| IBIS file 71v3578Z_bg.ibs created by s2ibis2 version 1.1
| North Carolina State University Electronics Research Laboratory  1995
[IBIS ver]   2.1
[File name]   71v3578z_bg.ibs
[File Rev]   1.1
[Date]   8/16/00
[Source]   Integrated Device Technology, Inc.
[Notes]   1. Temperatures: typ=25C, min=70C, max=0C 2. Cemos10_3v
   process. 3. Ramp rates based on 50 ohm load.
[Copyright]   Copyright 2000, Integrated Device Technology, Inc. Integrated
   Device Technology, Inc. ("IDT") hereby grants the user of this
   IBIS model a non-exclusive, nontransferable license to use
   this IBIS model under the following terms. The user is granted
   this license only to use the IBIS model and is not granted
   rights to sell, copy (except as needed to run the IBIS model),
   rent, lease or sub-license the IBIS model in whole or in part,
   or in modified form to anyone. The User may modify the IBIS
   model to suit its specific applications, but rights to
   derivative works and such modifications shall belong to IDT.
   This IBIS model is provided on an AS IS" basis and IDT makes
   absolutely no warranty with respect to the information
   contained herein. IDT DISCLAIMS AND CUSTOMER WAIVES ALL
   WARRANTIES, EXPRESS AND IMPLIED, INCLUDING WARRANTIES OF
   MERCHANTABILITY AND FITNESS FOR A PARTICULAR PURPOSE. THE
   ENTIRE RISK AS TO QUALITY AND PERFORMANCE IS WITH THE USER
   ACCORDINGLY, IN NO EVENT SHALL IDT BE LIABLE FOR ANY DIRECT OR
   INDIRECT DAMAGES, WHETHER IN CONTRACT OR TORT, INCLUDING ANY
   LOST PROFITS OR OTHER INCIDENTAL, CONSEQUENTIAL, EXEMPLARY, OR
   PUNITIVE DAMAGES ARISING OUT OF THE USE OR APPLICATION OF THE
   IBIS model. Further, IDT reserves the right to make changes
   without notice to any product herein to improve reliability,
   function, or design. IDT does not convey any license under
   patent rights or any other intellectual property rights,
   including those of third parties. IDT is not obligated to
   provide maintenance or support for the licensed IBIS model.
|   Component idt71V3578Z
[Component]   idt71V3578Z
[Manufacturer]   Integrated Device Technology
|   This component uses the 119 BGA package (BG)
[Package]
| variable   typ   min   max
R_pkg   328m   103m   556m
L_pkg   5.4nH   2.8nH   20.4nH
C_pkg   2.1pF   1.06pF   4.4pF
[Pin]  signal_name   model_name   R_pin   L_pin   C_pin
A1   VDDQ   POWER
A2   A6   INPAD_71V3578Z
A3   A4   INPAD_71V3578Z
A4   NADSP   INPAD_71V3578Z
A5   A8   INPAD_71V3578Z
A6   A16   INPAD_71V3578Z
A7   VDDQ   POWER
B1   NC   NC
B2   CS0   INPAD_71V3578Z
B3   A3   INPAD_71V3578Z
B4   NADSC   INPAD_71V3578Z
B5   A9   INPAD_71V3578Z
B6   NCS1   INPAD_71V3578Z
B7   NC   NC
C1   NC   NC
C2   A7   INPAD_71V3578Z
C3   A2   INPAD_71V3578Z
C4   VDD   POWER
C5   A13   INPAD_71V3578Z
C6   A17   INPAD_71V3578Z
C7   NC   NC
D1   IO8   IOPAD3578Z
D2   NC   NC
D3   VSS   GND
D4   NC   NC
D5   VSS   GND
D6   IO7   IOPAD3578Z
D7   NC   NC
E1   NC   NC
E2   IO9   IOPAD3578Z
E3   VSS   GND
E4   NCE   INPAD_71V3578Z
E5   VSS   GND
E6   NC   NC
E7   IO6   IOPAD3578Z
F1   VDDQ   POWER
F2   NC   NC
F3   VSS   GND
F4   NOE   INPAD_71V3578Z
F5   VSS   GND
F6   IO5   IOPAD3578Z
F7   VDDQ   POWER
G1   NC   NC
G2   IO10   IOPAD3578Z
G3   NBW2   INPAD_71V3578Z
G4   NADV   INPAD_71V3578Z
G5   VSS   GND
G6   NC   NC
G7   IO4   IOPAD3578Z
H1   IO11   IOPAD3578Z
H2   NC   NC
H3   VSS   GND
H4   NGW   INPAD_71V3578Z
H5   VSS   GND
H6   IO3   IOPAD3578Z
H7   NC   NC
J1   VDDQ   POWER
J2   VDD   POWER
J3   NC   NC
J4   VDD   POWER
J5   NC   NC
J6   VDD   POWER
J7   VDDQ   POWER
K1   NC   NC
K2   IO12   IOPAD3578Z
K3   VSS   GND
K4   CLK   INCLK_71V3578Z
K5   VSS   GND
K6   NC   NC
K7   IO2   IOPAD3578Z
L1   IO13   IOPAD3578Z
L2   NC   NC
L3   VSS   GND
L4   NC   NC
L5   NBW1   INPAD_71V3578Z
L6   IO1   IOPAD3578Z
L7   NC   NC
M1   VDDQ   POWER
M2   IO14   IOPAD3578Z
M3   VSS   GND
M4   NBWE   INPAD_71V3578Z
M5   VSS   GND
M6   NC   NC
M7   VDDQ   POWER
N1   IO15   IOPAD3578Z
N2   NC   NC
N3   VSS   GND
N4   A1   INPAD_71V3578Z
N5   VSS   GND
N6   IO0   IOPAD3578Z
N7   NC   NC
P1   NC   NC
P2   IOP2   IOPAD3578Z
P3   VSS   GND
P4   A0   INPAD_71V3578Z
P5   VSS   GND
P6   NC   NC
P7   IOP1   IOPAD3578Z
R1   NC   NC
R2   A5   INPAD_71V3578Z
R3   NLBO   INPAD_71V3578Z
R4   VDD   POWER
R5   VDD   POWER
R6   A12   INPAD_71V3578Z
R7   NC   NC
T1   NC   NC
T2   A10   INPAD_71V3578Z
T3   A15   INPAD_71V3578Z
T4   NC   NC
T5   A14   INPAD_71V3578Z
T6   A11   INPAD_71V3578Z
T7   ZZ   INPAD_71V3578Z
U1   VDDQ   POWER
U2   NC   NC
U3   NC   NC
U4   NC   NC
U5   NC   NC
U6   NC   NC
U7   VDDQ   POWER
U70   GNDQ   GND
| IOIN IOIN   dummy_model
| OC   OC   dummy_model
| IN   IN   dummy_model
| CLK  CLK   dummy_model
[Pin Mapping]  pulldown_ref   pullup_ref   gnd_clamp_ref   power_clamp_ref
A1   NC   EXTVDDQ
A2   EXTGNDQ   EXTVDDQ   EXTGND   EXTVDD
A3   EXTGNDQ   EXTVDDQ   EXTGND   EXTVDD
A4   EXTGNDQ   EXTVDDQ   EXTGND   EXTVDD
A5   EXTGNDQ   EXTVDDQ   EXTGND   EXTVDD
A6   EXTGNDQ   EXTVDDQ   EXTGND   EXTVDD
A7   NC   EXTVDDQ
B1   NC   NC   NC   NC
B2   EXTGNDQ   EXTVDDQ   EXTGND   EXTVDD
B3   EXTGNDQ   EXTVDDQ   EXTGND   EXTVDD
B4   EXTGNDQ   EXTVDDQ   EXTGND   EXTVDD
B5   EXTGNDQ   EXTVDDQ   EXTGND   EXTVDD
B6   EXTGNDQ   EXTVDDQ   EXTGND   EXTVDD
B7   NC   NC   NC   NC
C1   NC   NC   NC   NC
C2   EXTGNDQ   EXTVDDQ   EXTGND   EXTVDD
C3   EXTGNDQ   EXTVDDQ   EXTGND   EXTVDD
C4   NC   EXTVDD
C5   EXTGNDQ   EXTVDDQ   EXTGND   EXTVDD
C6   EXTGNDQ   EXTVDDQ   EXTGND   EXTVDD
C7   NC   NC   NC   NC
D1   EXTGNDQ   EXTVDDQ   EXTGND   EXTVDD
D2   NC   NC   NC   NC
D3   EXTGND   NC
D4   NC   NC   NC   NC
D5   EXTGND   NC
D6   EXTGNDQ   EXTVDDQ   EXTGND   EXTVDD
D7   NC   NC   NC   NC
E1   NC   NC   NC   NC
E2   EXTGNDQ   EXTVDDQ   EXTGND   EXTVDD
E3   EXTGND   NC
E4   EXTGNDQ   EXTVDDQ   EXTGND   EXTVDD
E5   EXTGND   NC
E6   NC   NC   NC   NC
E7   EXTGNDQ   EXTVDDQ   EXTGND   EXTVDD
F1   NC   EXTVDDQ
F2   NC   NC   NC   NC
F3   EXTGND   NC
F4   EXTGNDQ   EXTVDDQ   EXTGND   EXTVDD
F5   EXTGND   NC
F6   EXTGNDQ   EXTVDDQ   EXTGND   EXTVDD
F7   NC   EXTVDDQ
G1   NC   NC   NC   NC
G2   EXTGNDQ   EXTVDDQ   EXTGND   EXTVDD
G3   EXTGNDQ   EXTVDDQ   EXTGND   EXTVDD
G4   EXTGNDQ   EXTVDDQ   EXTGND   EXTVDD
G5   EXTGND   NC
G6   NC   NC   NC   NC
G7   EXTGNDQ   EXTVDDQ   EXTGND   EXTVDD
H1   EXTGNDQ   EXTVDDQ   EXTGND   EXTVDD
H2   NC   NC   NC   NC
H3   EXTGND   NC
H4   EXTGNDQ   EXTVDDQ   EXTGND   EXTVDD
H5   EXTGND   NC
H6   EXTGNDQ   EXTVDDQ   EXTGND   EXTVDD
H7   NC   NC   NC   NC
J1   NC   EXTVDDQ
J2   NC   EXTVDD
J3   NC   NC   NC   NC
J4   NC   EXTVDD
J5   NC   NC   NC   NC
J6   NC   EXTVDD
J7   NC   EXTVDDQ
K1   NC   NC   NC   NC
K2   EXTGNDQ   EXTVDDQ   EXTGND   EXTVDD
K3   EXTGND   NC
K4   EXTGNDQ   EXTVDDQ   EXTGND   EXTVDD
K5   EXTGND   NC
K6   NC   NC   NC   NC
K7   EXTGNDQ   EXTVDDQ   EXTGND   EXTVDD
L1   EXTGNDQ   EXTVDDQ   EXTGND   EXTVDD
L2   NC   NC   NC   NC
L3   EXTGND   NC
L4   NC   NC   NC   NC
L5   EXTGNDQ   EXTVDDQ   EXTGND   EXTVDD
L6   EXTGNDQ   EXTVDDQ   EXTGND   EXTVDD
L7   NC   NC   NC   NC
M1   NC   EXTVDDQ
M2   EXTGNDQ   EXTVDDQ   EXTGND   EXTVDD
M3   EXTGND   NC
M4   EXTGNDQ   EXTVDDQ   EXTGND   EXTVDD
M5   EXTGND   NC
M6   NC   NC   NC   NC
M7   NC   EXTVDDQ
N1   EXTGNDQ   EXTVDDQ   EXTGND   EXTVDD
N2   NC   NC   NC   NC
N3   EXTGND   NC
N4   EXTGNDQ   EXTVDDQ   EXTGND   EXTVDD
N5   EXTGND   NC
N6   EXTGNDQ   EXTVDDQ   EXTGND   EXTVDD
N7   NC   NC   NC   NC
P1   NC   NC   NC   NC
P2   EXTGNDQ   EXTVDDQ   EXTGND   EXTVDD
P3   EXTGND   NC
P4   EXTGNDQ   EXTVDDQ   EXTGND   EXTVDD
P5   EXTGND   NC
P6   NC   NC   NC   NC
P7   EXTGNDQ   EXTVDDQ   EXTGND   EXTVDD
R1   NC   NC   NC   NC
R2   EXTGNDQ   EXTVDDQ   EXTGND   EXTVDD
R3   EXTGNDQ   EXTVDDQ   EXTGND   EXTVDD
R4   NC   EXTVDD
R5   NC   EXTVDD
R6   EXTGNDQ   EXTVDDQ   EXTGND   EXTVDD
R7   NC   NC   NC   NC
T1   NC   NC   NC   NC
T2   NC   NC   NC   NC
T3   EXTGNDQ   EXTVDDQ   EXTGND   EXTVDD
T4   NC   NC   NC   NC
T5   EXTGNDQ   EXTVDDQ   EXTGND   EXTVDD
T6   NC   NC   NC   NC
T7   EXTGNDQ   EXTVDDQ   EXTGND   EXTVDD
U1   NC   EXTVDDQ
U2   NC   NC   NC   NC
U3   NC   NC   NC   NC
U4   NC   NC   NC   NC
U5   NC   NC   NC   NC
U6   NC   NC   NC   NC
U7   NC   EXTVDDQ
U70   EXTGNDQ   NC
| Models and submodels in the file (3): IOPAD3578Z (I/O), INCLK_71V3578Z (Input), INPAD_71V3578Z (Input)
